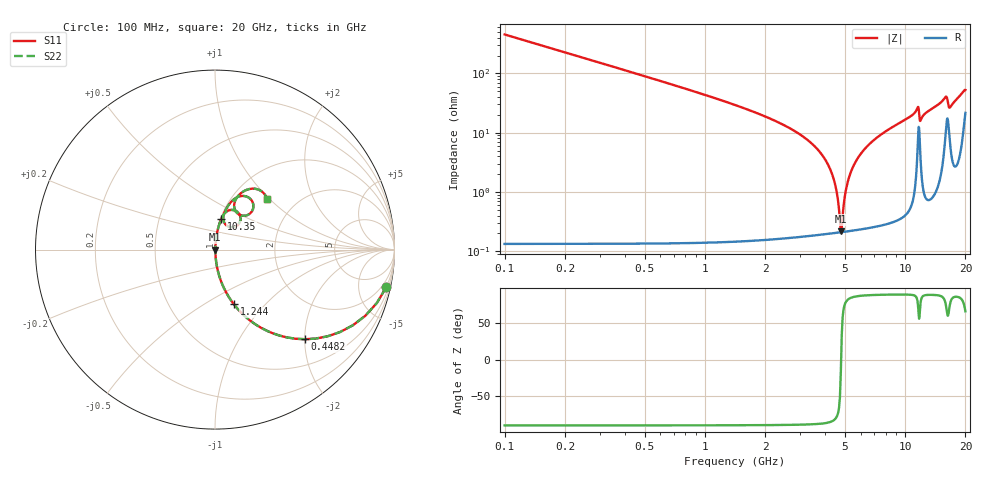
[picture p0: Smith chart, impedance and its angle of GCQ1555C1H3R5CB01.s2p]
!Murata Part Number: GCQ1555C1H3R5CB01
!These Parameters are Measured in Series Mode Connection
!Data Generated on Jan 08, 2026
!  o--ll--o
!Port1  Port2
!  o------o
!Operation Temp=25[degC], DC Bias Voltage=0[V]
!Freq. Start=100[MHz] Stop=20[GHz] 401[Steps]
# Hz S RI R 50
!Freq.(Hz) S11(Real) S11(Imag) S21(Real) S21(Imag) S12(Real) S12(Imag) S22(Real) S22(Imag)
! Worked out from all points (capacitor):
!   401 points, 100 MHz to 20 GHz, reference 50 ohm
!   read as one part in series: C = 3.5 pF near 199.5 MHz
!   lowest |Z| = 217 mohm at 4.777 GHz (marker M1)
!   series resonance near 4.792 GHz, so ESL is about 320 pH
!   S11 on the Smith chart (normalised r, x): 100 MHz: 1.00, -9.09; 448.2 MHz: 1.00, -2.01; 1.244 GHz: 1.00, -0.68; 10.35 GHz: 1.01, +0.35; 20 GHz: 1.43, +0.96
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1e8  0.9538 -0.2098  0.0462 0.2098  0.0462 0.2098  0.9538 -0.2098
4.4825e8  0.5028 -0.4993  0.4972 0.4993  0.4972 0.4993  0.5028 -0.4993
7.965e8  0.2362 -0.4235  0.7638 0.4235  0.7638 0.4235  0.2362 -0.4235
1.24425e9  0.1051 -0.3047  0.8949 0.3047  0.8949 0.3047  0.1051 -0.3047
3.43325e9  0.00597 -0.0642  0.994 0.0642  0.994 0.0642  0.00597 -0.0642
4.32875e9  0.00237 -0.0194  0.9976 0.0194  0.9976 0.0194  0.00237 -0.0194
4.52775e9  0.00215 -0.0108  0.9978 0.0108  0.9978 0.0108  0.00215 -0.0108
4.7765e9  0.00208 -0.000596  0.9979 0.000596  0.9979 0.000596  0.00208 -0.000596
4.876e9  0.00211 0.00334  0.9979 -0.00334  0.9979 -0.00334  0.00211 0.00334
5.12475e9  0.00232 0.0129  0.9977 -0.0129  0.9977 -0.0129  0.00232 0.0129
5.42325e9  0.00277 0.0237  0.9972 -0.0237  0.9972 -0.0237  0.00277 0.0237
5.9705e9  0.00413 0.0425  0.9959 -0.0425  0.9959 -0.0425  0.00413 0.0425
6.7665e9  0.00711 0.0677  0.9929 -0.0677  0.9929 -0.0677  0.00711 0.0677
1.005e10  0.0309 0.1612  0.9691 -0.1612  0.9691 -0.1612  0.0309 0.1612
1.03485e10  0.0346 0.1704  0.9654 -0.1704  0.9654 -0.1704  0.0346 0.1704
1.15425e10  0.104 0.2206  0.896 -0.2206  0.896 -0.2206  0.104 0.2206
1.19405e10  0.0565 0.1425  0.9435 -0.1425  0.9435 -0.1425  0.0565 0.1425
1.338325e10  0.0626 0.2275  0.9374 -0.2275  0.9374 -0.2275  0.0626 0.2275
1.59205e10  0.1887 0.289  0.8113 -0.289  0.8113 -0.289  0.1887 0.289
1.67165e10  0.1181 0.2098  0.8819 -0.2098  0.8819 -0.2098  0.1181 0.2098
1.89055e10  0.1826 0.3351  0.8174 -0.3351  0.8174 -0.3351  0.1826 0.3351
2e10  0.2885 0.2811  0.7115 -0.2811  0.7115 -0.2811  0.2885 0.2811
